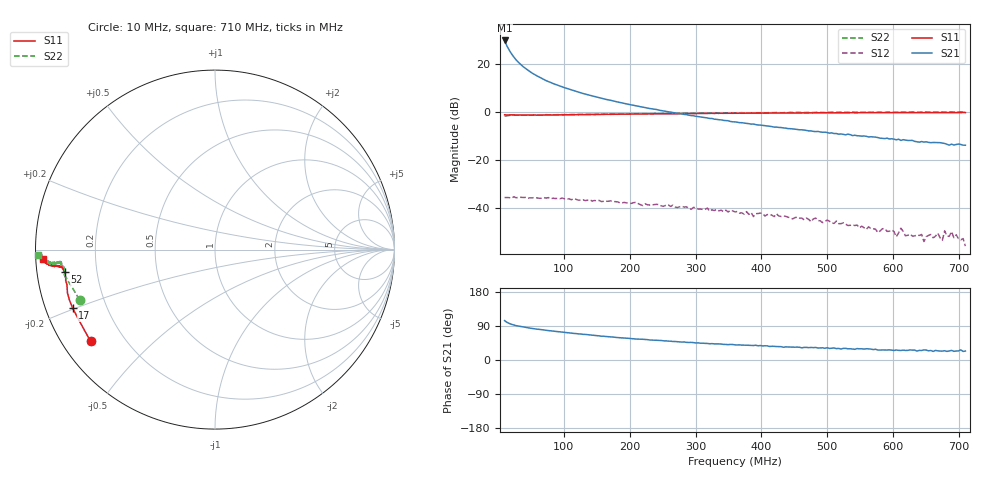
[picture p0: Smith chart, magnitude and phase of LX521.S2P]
!  POLYFET RF DEVICES
!  LX521
!  S PARAMETERS
!  VDS=12.5V, IDQ=800mA
! Date: Wed Jul 16 09:24:44 2003
# MHZ S MA R 50
! Freq=Mhz Mag[s11] Ang[s11] Mag[s21] Ang[s21] Mag[s12] Ang[s12] Mag[s22] Ang[s22]
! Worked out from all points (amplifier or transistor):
!   201 points, 10 MHz to 710 MHz, reference 50 ohm
!   highest |S21| = 29.7 dB at 10 MHz (marker M1)
!   |S21| within 3 dB of that: start of sweep to 14.93 MHz
!   unconditionally stable (mu >= 1): 527.3 MHz to 536.1 MHz; 564 MHz to 614.8 MHz; 630.5 MHz to 703 MHz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
!   at 125.5 MHz: K = 0.27, MSG = 22.4 dB, |S12| = -36.9 dB
!   at 360 MHz: K = 0.75, MSG = 18.8 dB, |S12| = -41.8 dB
!   at 710 MHz: K = 2.73, MAG = 13.8 dB, |S12| = -56.1 dB
!   S11 on the Smith chart (normalised r, x): 10 MHz: 0.08, -0.33; 17 MHz: 0.08, -0.20; 52 MHz: 0.08, -0.07; 710 MHz: 0.02, -0.03
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10  0.8613 -143.6  30.54 103.9  0.01622 16.1  0.8049 -159.7
13.5  0.854 -152.3  23.47 99.4  0.01622 11.2  0.8217 -164.8
17  0.8577 -157.7  19.2 96.5  0.01613 8.6  0.8347 -167.4
20.5  0.8583 -161.1  16.08 94.1  0.01573 4.4  0.8433 -169.4
24  0.8567 -163.7  13.81 92.5  0.0168 4.2  0.8508 -170.5
27.5  0.8514 -165.3  12.01 90.7  0.01602 3.5  0.8447 -171.4
31  0.8474 -166.8  10.7 89.5  0.01639 0.4  0.8446 -172.9
38  0.8471 -169.0  8.726 87.0  0.01629 -2.6  0.856 -173.5
45  0.8507 -170.5  7.4 84.9  0.01567 -1.8  0.8557 -174.1
52  0.8461 -171.4  6.35 83.2  0.01595 -2.6  0.8578 -174.9
66  0.8518 -172.3  4.962 80.0  0.01566 -8.9  0.8498 -175.0
83.5  0.8509 -173.3  3.868 76.3  0.01573 -10.1  0.8634 -175.4
101  0.8586 -173.6  3.165 72.8  0.01526 -11.6  0.866 -175.7
129  0.8718 -173.6  2.395 67.7  0.01458 -16.7  0.8732 -175.4
181.5  0.8831 -174.1  1.595 59.2  0.01318 -25.1  0.9017 -175.3
244.5  0.9034 -174.3  1.075 51.6  0.01146 -28.3  0.913 -175.3
360  0.9263 -174.8  0.6125 39.9  0.00813 -31.2  0.9414 -175.7
479  0.946 -175.7  0.3888 32.6  0.00579 -28.4  0.9595 -176.7
594.5  0.9556 -176.2  0.2701 26.9  0.00321 -20.1  0.9767 -178.4
647  0.9547 -176.7  0.2326 26.7  0.00196 -1.7  0.9782 -177.9
689  0.9567 -176.9  0.2106 25.3  0.00317 -1.2  0.9822 -178.3
710  0.9603 -177.0  0.1997 23.7  0.00157 -7.2  0.9852 -178.3
